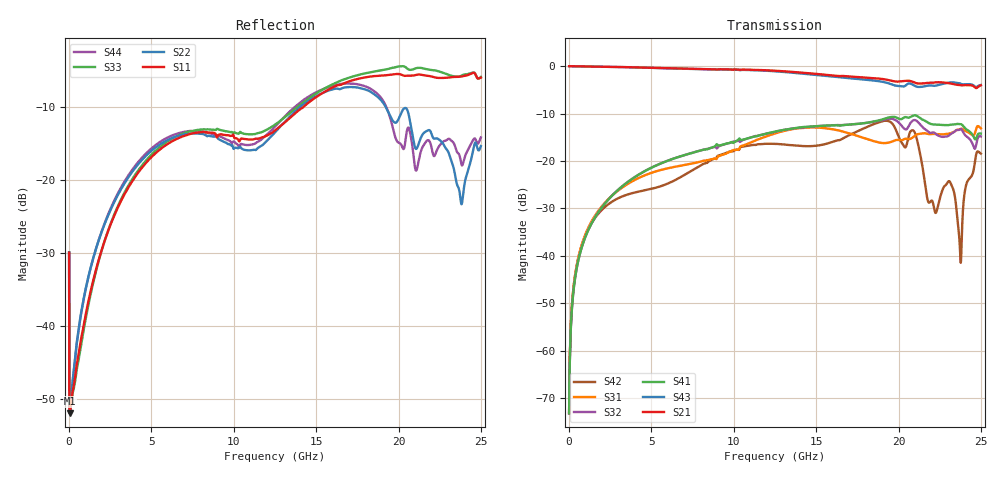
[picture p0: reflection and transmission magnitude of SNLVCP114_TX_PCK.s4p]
! Touchstone Ver. 1.0
! Mon Jun 18 17:08:35 2012
! Number of ports is 4
# Hz	S	MA	R	50.000000
! SCATTERING PARAMETERS  :
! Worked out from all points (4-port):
!   2501 points, 1 MHz to 25 GHz, reference 50 ohm
!   strongest paths, dB at 1 MHz, 6.251 GHz, 12.5 GHz, 18.75 GHz, 25 GHz:
!     S21: 0.0, -0.5, -1.0, -2.6, -4.1
!     S43: 0.0, -0.5, -1.1, -3.2, -4.0
!     S41: -73.2, -19.6, -13.8, -11.5, -14.2
!     S32: -73.2, -19.6, -13.8, -11.6, -14.8
!     S31: -73.1, -21.3, -14.2, -16.0, -13.1
!     S42: -73.1, -24.3, -16.4, -11.9, -18.5
!   lowest |S11| = -51.9 dB at 41 MHz (marker M1), VSWR 1.01, Z = 50.2 - j0.0655 ohm
!   |S11| at or under -10 dB: start of sweep to 14.25 GHz
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1000000  0.03182 -84.3  0.9973 1.8  0.000221 5.5  0.0002198 -174.5
         0.9973 1.8  0.03182 -84.3  0.0002198 -174.5  0.0002209 5.5
         0.000221 5.5  0.0002198 -174.5  0.03182 -84.2  0.9973 1.8
         0.0002198 -174.5  0.0002209 5.5  0.9973 1.8  0.03182 -84.2
4.1e7  0.002532 -14.9  0.9974 -0.8  0.0007958 66.9  0.0007462 -114.5
       0.9974 -0.8  0.00256 -15.1  0.0007462 -114.5  0.0007929 65.9
       0.0007958 66.9  0.0007462 -114.5  0.00254 -14.0  0.9974 -0.8
       0.0007462 -114.5  0.0007929 65.9  0.9974 -0.8  0.002569 -14.2
9.91e8  0.0118 -115.2  0.9907 -18.1  0.01691 83.8  0.01592 -108.6
        0.9907 -18.1  0.01768 -61.2  0.01593 -108.6  0.01651 59.0
        0.01691 83.8  0.01593 -108.6  0.01096 -118.0  0.9907 -18.1
        0.01592 -108.6  0.01651 59.0  0.9907 -18.1  0.01745 -58.1
4.501e9  0.124 133.7  0.9646 -80.9  0.06958 68.4  0.07656 -174.2
         0.9646 -80.9  0.1396 -114.7  0.07671 -174.3  0.04871 -60.5
         0.06958 68.4  0.07671 -174.3  0.1286 131.0  0.9634 -81.2
         0.07656 -174.2  0.04871 -60.5  0.9634 -81.2  0.1447 -113.4
1.4551e10  0.3379 80.0  0.8404 100.1  0.2252 40.3  0.23 -8.4
           0.8404 100.1  0.3474 -78.3  0.2293 -8.6  0.1432 -82.5
           0.2252 40.3  0.2293 -8.6  0.3601 76.0  0.8207 98.9
           0.23 -8.4  0.1432 -82.5  0.8207 98.9  0.3713 -78.9
2.3741e10  0.5079 27.4  0.6287 -56.2  0.217 28.5  0.245 165.7
           0.6287 -56.2  0.07754 8.3  0.2159 176.1  0.01085 -51.4
           0.217 28.5  0.2159 176.1  0.5097 19.4  0.6564 -51.7
           0.245 165.7  0.01085 -51.4  0.6564 -51.7  0.1411 62.0
2.5001e10  0.4994 25.5  0.6268 -74.6  0.221 18.9  0.1943 154.3
           0.6268 -74.6  0.17 -28.1  0.1814 164.0  0.1195 43.3
           0.221 18.9  0.1814 164.0  0.5051 17.9  0.6323 -71.3
           0.1943 154.3  0.1195 43.3  0.6323 -71.3  0.1949 -8.8
